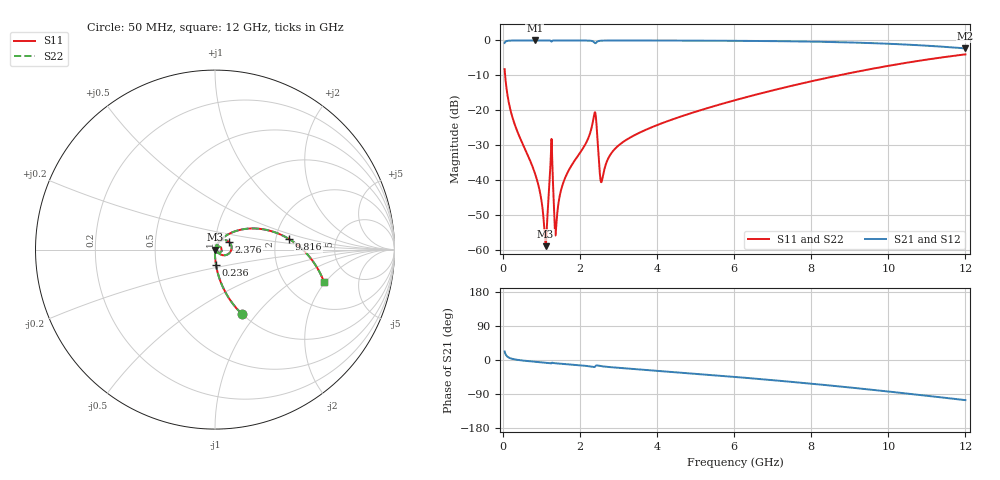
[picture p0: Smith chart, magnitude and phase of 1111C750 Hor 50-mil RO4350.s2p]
# GHz S MA R 50
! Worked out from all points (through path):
!   11951 points, 50 MHz to 12 GHz, reference 50 ohm
!   highest |S21| = -0.01 dB at 831 MHz (marker M1); lowest = -2.3 dB at 12 GHz (marker M2)
!   group delay of S21, straight-line fit = 24.7 ps
!   lowest |S11| = -58.8 dB at 1.114 GHz (marker M3), VSWR 1.00, Z = 50.1 - j0.0193 ohm
!   |S11| at or under -10 dB: 63.23 MHz to 8.709 GHz (8.646 GHz wide, 197 % of centre)
!   |S22| runs from -58.8 to -4.0 dB; largest |S21 - S12| = 0
!   S11 on the Smith chart (normalised r, x): 50 MHz: 1.00, -0.84; 236 MHz: 1.00, -0.17; 2.376 GHz: 1.17, +0.10; 9.816 GHz: 2.36, +0.34; 12 GHz: 3.22, -1.91
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0.05  0.3887 -67.4  0.9211 22.6  0.9211 22.6  0.3887 -67.4
0.236  0.08583 -86.2  0.9958 3.4  0.9958 3.4  0.08583 -86.2
0.831  0.0129 -90.8  0.999 -4.5  0.999 -4.5  0.0129 -90.8
0.968  0.006756 -87.8  0.999 -5.7  0.999 -5.7  0.006756 -87.8
1.114  0.001149 -9.6  0.9988 -7.0  0.9988 -7.0  0.001149 -9.6
1.154  0.002669 52.3  0.9986 -7.4  0.9986 -7.4  0.002669 52.3
1.25  0.02394 46.3  0.9861 -9.0  0.9861 -9.0  0.02394 46.3
1.284  0.02062 -57.0  0.9865 -7.2  0.9865 -7.2  0.02062 -57.0
1.347  0.002373 -45.3  0.998 -8.4  0.998 -8.4  0.002373 -45.3
1.388  0.002183 39.4  0.9985 -8.9  0.9985 -8.9  0.002183 39.4
1.587  0.0098 72.2  0.9986 -10.6  0.9986 -10.6  0.0098 72.2
2.042  0.02656 71.2  0.9975 -14.4  0.9975 -14.4  0.02656 71.2
2.376  0.08933 28.8  0.9374 -18.7  0.9374 -18.7  0.08933 28.8
2.525  0.01168 -20.9  0.9882 -15.8  0.9882 -15.8  0.01168 -20.9
2.572  0.00984 26.1  0.9926 -16.5  0.9926 -16.5  0.00984 26.1
2.96  0.03002 65.4  0.9971 -20.2  0.9971 -20.2  0.03002 65.4
4.034  0.06258 59.6  0.9958 -28.6  0.9958 -28.6  0.06258 59.6
6.025  0.1399 44.3  0.9873 -44.7  0.9873 -44.7  0.1399 44.3
8.017  0.2617 26.6  0.9614 -62.7  0.9614 -62.7  0.2617 26.6
9.816  0.4155 8.3  0.9049 -81.1  0.9049 -81.1  0.4155 8.3
10.009  0.434 6.2  0.8961 -83.3  0.8961 -83.3  0.434 6.2
12  0.6321 -16.4  0.7689 -105.9  0.7689 -105.9  0.6321 -16.4
